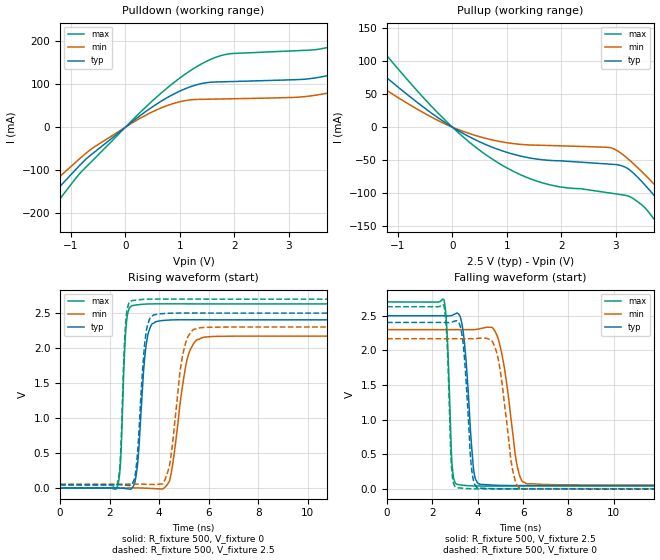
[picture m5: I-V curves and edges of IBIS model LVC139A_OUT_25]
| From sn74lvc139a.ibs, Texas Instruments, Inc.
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[Model]   LVC139A_OUT_25
Model_type  Output
Vref =   0
Rref =   500
Cref =   30p
Vmeas =   1.25
| variable   typ   min   max
C_comp   5.61pF   2.74pF   10.29pF
| C_pullup   4.78pF   3.34pF   5.77pF
| C_pulldown   6.43pF   2.74pF   10.29pF
[Temperature Range]   40   100   -40
| Ambient temperature   25   85   -40
[Voltage range]   2.5   2.3   2.7
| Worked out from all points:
|   slope of the pulldown table from 0 to 0.375 V, typ, clamps not added: 10.3 ohm
|   slope of the pullup table from 0 to 0.375 V, typ, clamps not added: 21.6 ohm
|   rising waveform, R_fixture 500, V_fixture 0: 20-80 % time 272ps typ, 482ps min, 163ps max; typ from 0 V to 2.4 V
|   falling waveform, R_fixture 500, V_fixture 2.5: 20-80 % time 306ps typ, 531ps min, 169ps max; typ from 2.5 V to 0.047 V
|   rising waveform, R_fixture 500, V_fixture 2.5: 20-80 % time 266ps typ, 432ps min, 161ps max; typ from 0.047 V to 2.5 V
|   falling waveform, R_fixture 500, V_fixture 0: 20-80 % time 270ps typ, 477ps min, 159ps max; typ from 2.4 V to 0 V
[Pulldown]
| LVC139A_OUT_25
|   Voltage   I(typ)   I(min)   I(max)
-5.5V     -638.7mA   -541.9mA   -776.5mA
-2.375V   -290.9mA   -241.3mA   -354.3mA
-1.83V    -221.7mA   -184.1mA   -269mA
-1.56V    -186.2mA   -154.6mA   -225.5mA
425mV     41.15mA    31.34mA    53.1mA
1.2V      94.47mA    63.65mA    132.4mA
1.85V     105.9mA    65.91mA    169.7mA
4.065V    132.3mA    89.58mA    200.1mA
4.655V    159.8mA    112.1mA    235.8mA
5.895V    236.1mA    174.2mA    338.5mA
6.925V    311.2mA    236.1mA    438.9mA
11V       662.3mA    531.1mA    902mA
[Pullup]
| LVC139A_OUT_25
|   Voltage   I(typ)   I(min)   I(max)
-5.5V     427.6mA    339.5mA    593.6mA
-2.835V   198.7mA    153.2mA    281.1mA
-2.31V    157mA      119.9mA    223.4mA
-1.655V   107.3mA    80.76mA    154.1mA
720mV     -30.07mA   -19.18mA   -47.78mA
1.685V    -49.79mA   -27.64mA   -85.3mA
2.92V     -56.36mA   -31.51mA   -100.3mA
3.28V     -66.47mA   -52mA      -106.4mA
3.875V    -120.3mA   -101.2mA   -159.2mA
4.225V    -156.2mA   -132.5mA   -202mA
4.505V    -185.8mA   -158.3mA   -237.6mA
11V       -923.8mA   -794mA     -1.133A
[Ramp]
| LVC139A_OUT_25
| variable   typ   min   max
dV/dt_r   1.45/2.90E-10   1.31/4.97E-10   1.59/1.69E-10
dV/dt_f   1.50/3.28E-10   1.37/5.58E-10   1.62/1.79E-10
R_load = 500
[Rising Waveform]
| LVC139A_OUT_25
R_fixture =   500
C_fixture =   0
L_fixture =   0
V_fixture =   0
V_fixture_min = 0
V_fixture_max = 0
|   Time   V(typ)   V(min)   V(max)
0s        26.07pV    2.337nV    1.74nV
2.295ns   349.2uV    -6.131uV   553.6uV
2.445ns   -1.774mV   -25.79uV   419.2mV
2.66ns    -9.632mV   49.81uV    2.3V
2.92ns    4.971mV    326.8uV    2.609V
3.51ns    2.128V     -3.638mV   2.63V
4.055ns   2.391V     -13.81mV   2.633V
5.17ns    2.405V     1.895V     2.632V
5.82ns    2.405V     2.156V     2.632V
50ns      2.404V     2.169V     2.632V
[Falling Waveform]
| LVC139A_OUT_25
R_fixture =   500
C_fixture =   0
L_fixture =   0
V_fixture =   2.5
V_fixture_min = 2.3
V_fixture_max = 2.7
|   Time   V(typ)   V(min)   V(max)
0s        2.5V       2.3V       2.7V
2.5ns     2.5V       2.3V       2.738V
2.875ns   2.508V     2.3V       321.8mV
3.17ns    2.52V      2.3V       58.6mV
3.82ns    274.1mV    2.3V       42.44mV
4.14ns    64.7mV     2.317V     40.95mV
4.905ns   50.83mV    2.164V     40.38mV
5.74ns    47.47mV    329.9mV    40.58mV
6.205ns   47.26mV    69.83mV    40.65mV
50ns      47.3mV     55.16mV    40.72mV
[Rising Waveform]
| LVC139A_OUT_25
R_fixture =   500
C_fixture =   0
L_fixture =   0
V_fixture =   2.5
V_fixture_min = 2.3
V_fixture_max = 2.7
|   Time   V(typ)   V(min)   V(max)
0s        47.3mV     55.16mV    40.72mV
2.29ns    47.59mV    55.16mV    42.76mV
2.65ns    39.8mV     55.21mV    2.38V
2.91ns    60.35mV    55.42mV    2.68V
3.47ns    2.223V     52.7mV     2.698V
3.945ns   2.486V     52.29mV    2.701V
4.415ns   2.498V     320.5mV    2.701V
5.05ns    2.501V     2.053V     2.7V
5.655ns   2.501V     2.291V     2.7V
50ns      2.5V       2.3V       2.7V
[Falling Waveform]
| LVC139A_OUT_25
R_fixture =   500
C_fixture =   0
L_fixture =   0
V_fixture =   0
V_fixture_min = 0
V_fixture_max = 0
|   Time   V(typ)   V(min)   V(max)
0s        2.404V     2.169V     2.632V
2.5ns     2.404V     2.169V     2.656V
2.85ns    2.408V     2.169V     286.6mV
3.135ns   2.413V     2.169V     14.63mV
3.75ns    237.1mV    2.169V     1.532mV
4.09ns    8.69mV     2.177V     87.02uV
4.84ns    1.783mV    1.963V     -292.4uV
5.535ns   61.51uV    281mV      -124.5uV
6.015ns   -56.36uV   -4.524mV   -53.12uV
50ns      -4.283nV   -152.1pV   -377.6pV
